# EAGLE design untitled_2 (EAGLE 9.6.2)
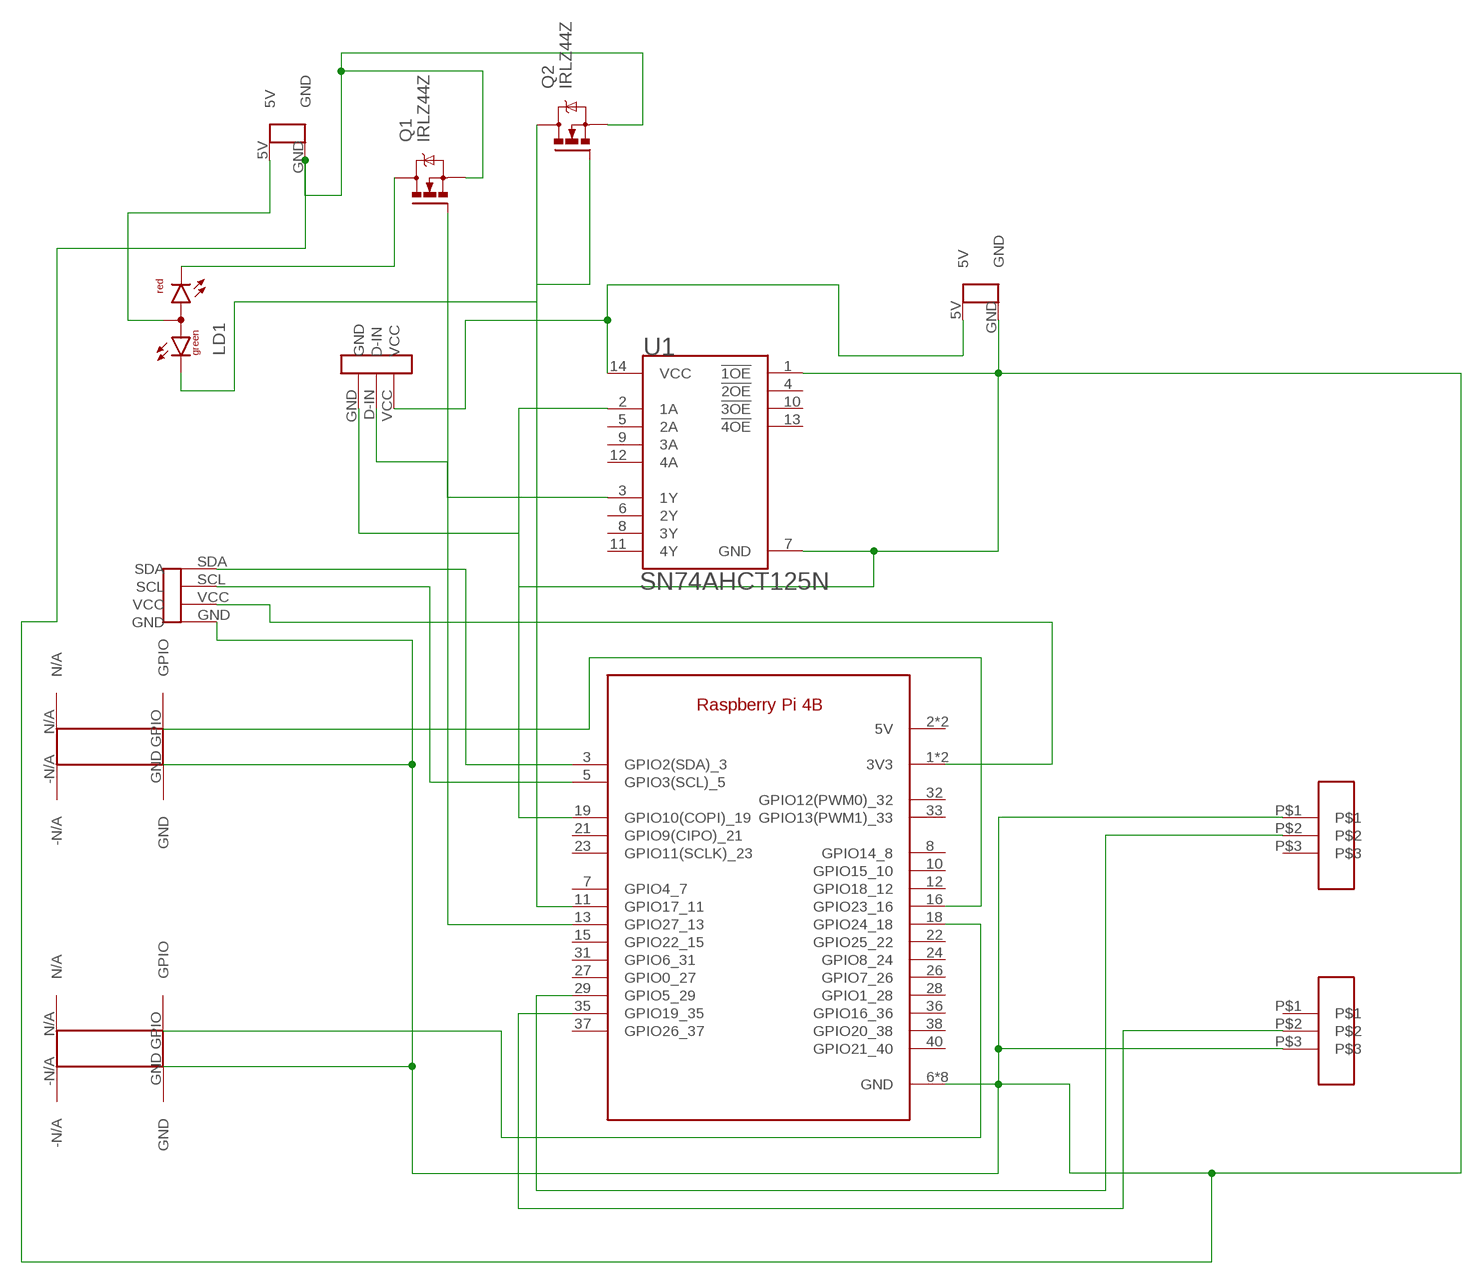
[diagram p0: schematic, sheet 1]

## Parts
LD1  DUOLED-RG-A  [DUOLED-A-5MM]
Q1  IRLZ44Z  [TO220BH]
Q2  IRLZ44Z  [TO220BH]
U1  TEXAS_INSTRUMENTS_SN74AHCT125NTEXAS_INSTRUMENTS_SN74AHCT125N_0_0  [TEXAS_INSTRUMENTS_SN74AHCT125N_0]
U$1  RASPBERRY_PI_4  [RASPI_4B]
U$2  G13-SW  [G13-SW]
U$3  G13-SW  [G13-SW]
U$4  LIGHTSENSOR-PO  [LIGHTSENSOR-IO]
U$5  LED-STRIP-PO  [LED-STRIP-PO]
U$6  G13-BUTTON  [G13-BUTTON]
U$7  G13-BUTTON  [G13-BUTTON]
U$8  G13-BATTERY  [G13-BATTERY]
U$10  G13-BATTERY  [G13-BATTERY]

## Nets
GND: Q1.S Q2.S U1.1(!1OE!) U1.7(GND) U$1.6(GND) U$1.9(GND) U$1.14(GND) U$1.20(GND) U$1.25(GND) U$1.30(GND) U$1.34(GND) U$1.39(GND) U$2.P$1 U$3.P$3 U$4.GND U$5.GND U$6.GND U$7.GND U$8.GND U$10.GND
N$1: U$1.3(GPIO2(SDA)_3) U$4.SDA
N$2: U$1.5(GPIO3(SCL)_5) U$4.SCL
N$3: U$1.1(3V3) U$1.17(3V3) U$4.VCC
N$4: LD1.CR Q1.D
N$5: U$1.16(GPIO23_16) U$6.GPIO
N$6: U$1.18(GPIO24_18) U$7.GPIO
N$7: U$1.29(GPIO5_29) U$2.P$2
N$8: U$1.35(GPIO19_35) U$3.P$2
N$9: U1.2(1A) U$1.19(GPIO10(COPI)_19)
N$10: U1.3(1Y) U$5.D-IN
N$11: U1.14(VCC) U$5.VCC U$8.5V
N$12: LD1.CX(CG) Q2.D
N$13: LD1.A U$10.5V
N$14: Q2.G U$1.11(GPIO17_11)
N$15: Q1.G U$1.13(GPIO27_13)
Unconnected: U1.4(!2OE!) U1.5(2A) U1.6(2Y) U1.8(3Y) U1.9(3A) U1.10(!3OE!) U1.11(4Y) U1.12(4A) U1.13(!4OE!) U$1.2(5V) U$1.4(5V) U$1.7(GPIO4_7) U$1.8(GPIO14_8) U$1.10(GPIO15_10) U$1.12(GPIO18_12) U$1.15(GPIO22_15) U$1.21(GPIO9(CIPO)_21) U$1.22(GPIO25_22) U$1.23(GPIO11(SCLK)_23) U$1.24(GPIO8_24) U$1.26(GPIO7_26) U$1.27(GPIO0_27) U$1.28(GPIO1_28) U$1.31(GPIO6_31) U$1.32(GPIO12(PWM0)_32) U$1.33(GPIO13(PWM1)_33) U$1.36(GPIO16_36) U$1.37(GPIO26_37) U$1.38(GPIO20_38) U$1.40(GPIO21_40) U$2.P$3 U$3.P$1 U$6.-N/A U$6.N/A U$7.-N/A U$7.N/A

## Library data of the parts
LD1 = led:DUOLED-RG-A: DUO LED 2 colors (red/green), 5 mm, round, common Anode www.ligitek.com or other producers.
Q1 Q2 = transistor-power:IRLZ44Z: N-Channel HEXFET® Power MOSFET Logic Level AUTOMOTIVE MOSFET Source: http://www.irf.com/product-info/datasheets/data/irlz44zpbf.pdf
U1 = Texas Instruments - SN74AHCT125N:TEXAS_INSTRUMENTS_SN74AHCT125N: QUADRUPLE BUS BUFFER GATES WITH 3-STATE OUTPUTS; CENTROID_NOT_SPECIFIED: No; DATASHEET: http://www.ti.com/lit/ds/symlink/sn74ahct125.pdf; DIGIKEY_DESCRIPTION: IC BUS BUFFER TRI-ST QD 14DIP; DIGIKEY_PART_NUMBER: 296-4655-5-ND; IPC_LAND_PATTERN_NAME: DIP794W46P254L1930H508Q14; LEAD_FREE: yes; MF: Texas Instruments; MOUSER_PART_NUMBER: 595-SN74AHCT125N; MPN: SN74AHCT125N; PACKAGE: PDIP-14; PREFIX: U; ROHS: yes; TEMPERATURE_RANGE_HIGH: +125°C; TEMPERATURE_RANGE_LOW: -40°C
U$1 = raspberryPi4:RASPBERRY_PI_4
U$2 U$3 = raspberryPi4:G13-SW
U$4 = raspberryPi4:LIGHTSENSOR-PO
U$5 = raspberryPi4:LED-STRIP-PO
U$6 U$7 = raspberryPi4:G13-BUTTON
U$8 U$10 = raspberryPi4:G13-BATTERY

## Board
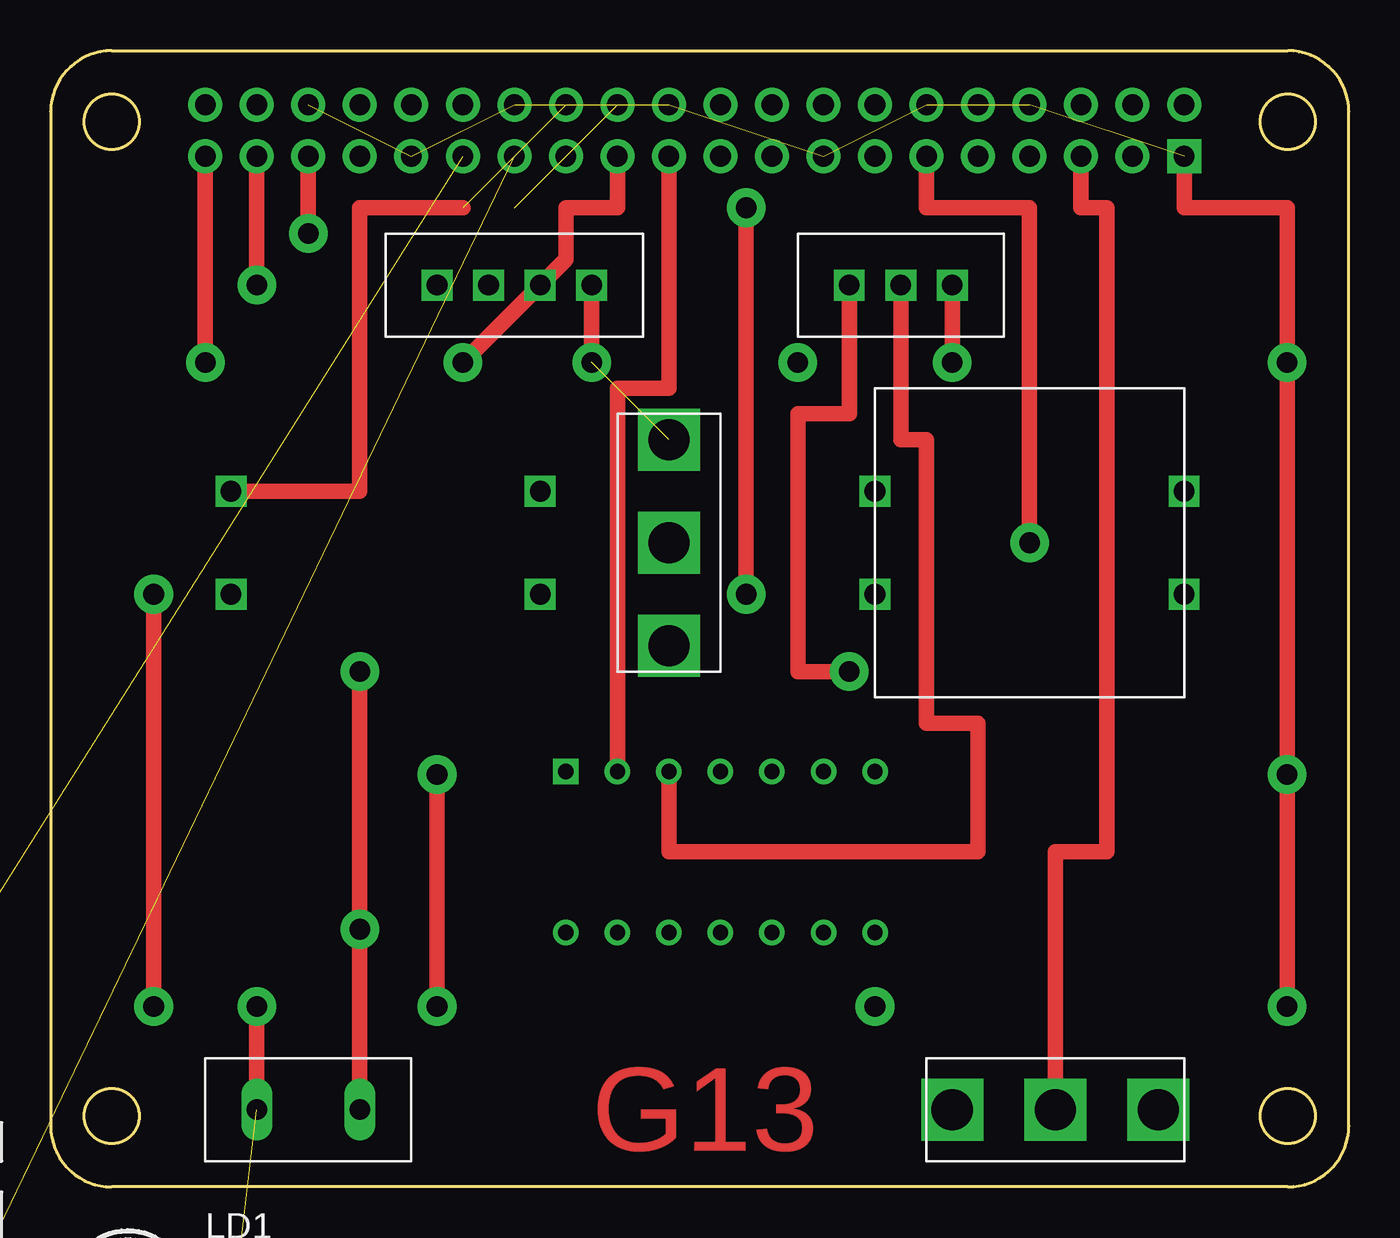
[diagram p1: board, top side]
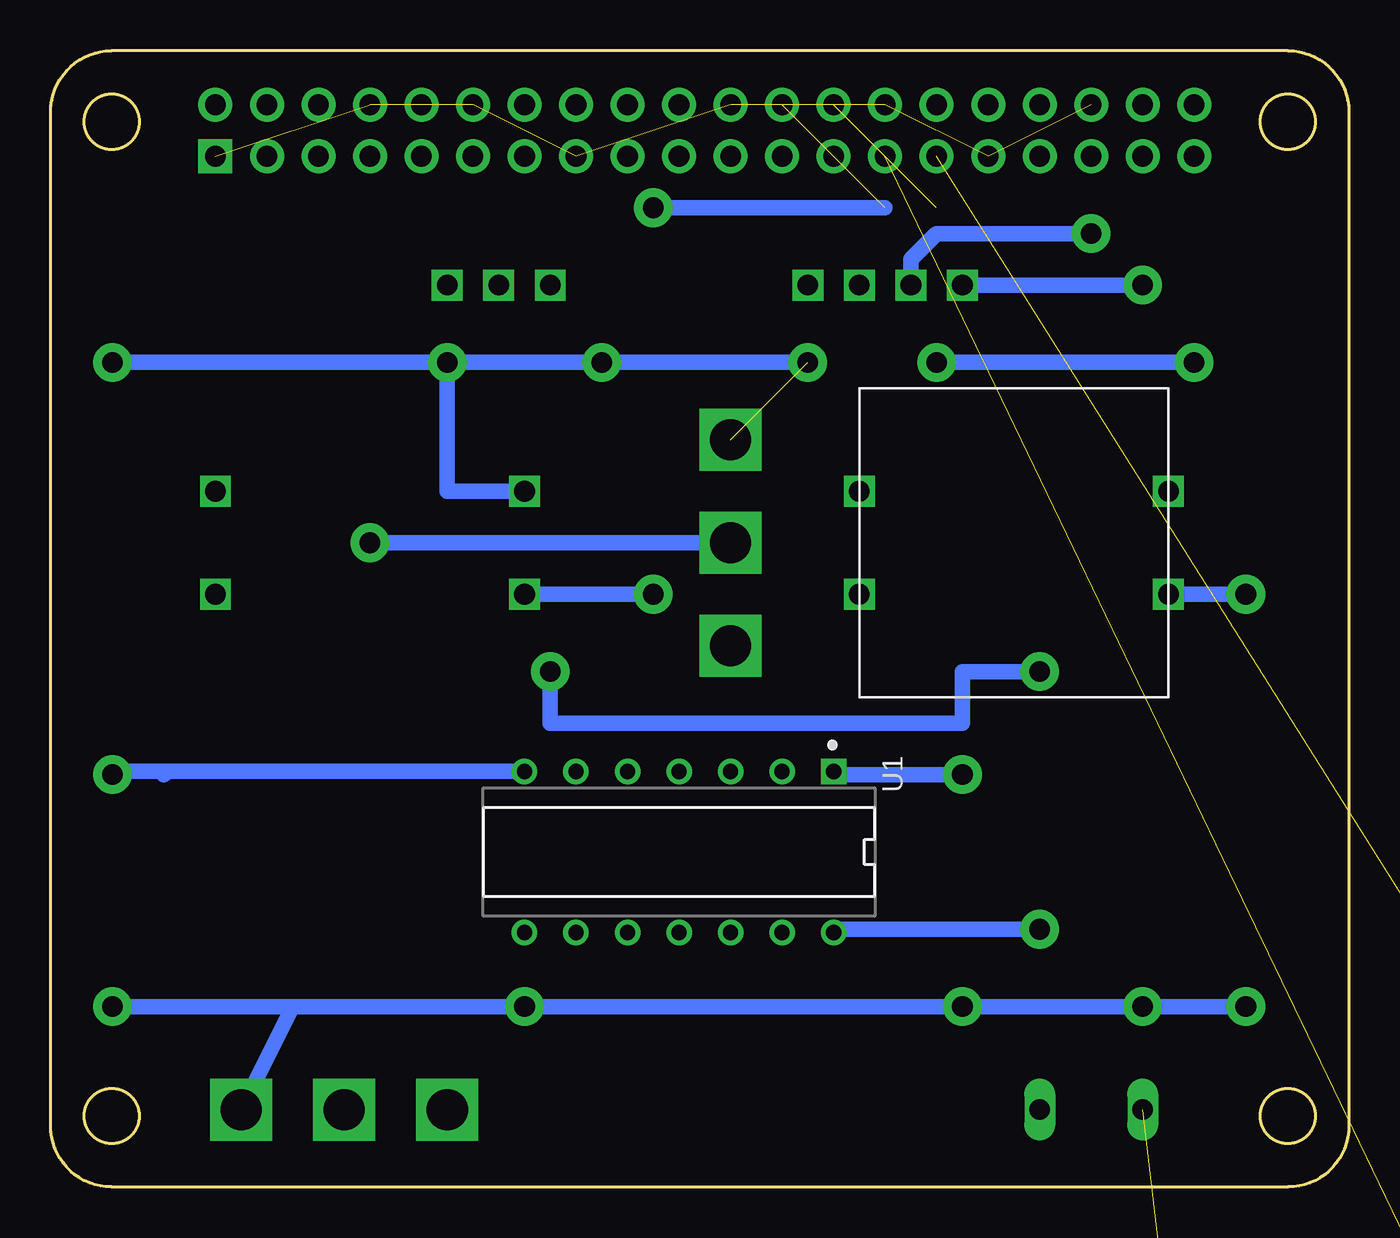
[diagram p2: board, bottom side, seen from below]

Size 64 x 56 mm. Coordinates in mm from the lower left corner, seen from the top.
Outline: 64,3 64,53 arc90 61,56 3,56 arc90 0,53 0,3 arc90 3,0 61,0 arc90 64,3
Outline: circle at 61,52.5 radius 1.35
Outline: circle at 61,3.5 radius 1.35
Outline: circle at 3,52.5 radius 1.35
Outline: circle at 3,3.5 radius 1.35
Copper layers (1*16): Top 0.035mm / dielectric 1.5mm / Bottom 0.035mm
Design rules "default": minimum track width 6mil, minimum drill 0.35mm, track to track 6mil, track to pad 6mil, pad to pad 6mil, via to via 6mil, smd to smd 6mil, copper to edge 40mil, drill to drill 6mil, minimum pad ring 10mil, minimum via ring 8mil, stop-mask expansion 4mil, vias tented up to drill 0mil, thermal gap 10mil

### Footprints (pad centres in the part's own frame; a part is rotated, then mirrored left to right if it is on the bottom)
DUOLED-A-5MM = drill 0.813 long: A 0,0; CR 2.54,0; CX -2.54,0
TO220BH = drill 1.118 long: D 0,-6.35; G -2.54,-6.35; S 2.54,-6.35 | hole 3.302: 0,11.176
TEXAS_INSTRUMENTS_SN74AHCT125N_0 = drill 0.75 pad 1.25 square: 1 -3.97,7.62 | drill 0.75 pad 1.25: 2 -3.97,5.08; 3 -3.97,2.54; 4 -3.97,0; 5 -3.97,-2.54; 6 -3.97,-5.08; 7 -3.97,-7.62; 8 3.97,-7.62; 9 3.97,-5.08; 10 3.97,-2.54; 11 3.97,0; 12 3.97,2.54; 13 3.97,5.08; 14 3.97,7.62
RASPI_4B = drill 1.016 pad 1.676: 1 -24.13,-1.27; 2 -24.13,1.27; 3 -21.59,-1.27; 4 -21.59,1.27; 5 -19.05,-1.27; 6 -19.05,1.27; 7 -16.51,-1.27; 8 -16.51,1.27; 9 -13.97,-1.27; 10 -13.97,1.27; 11 -11.43,-1.27; 12 -11.43,1.27; 13 -8.89,-1.27; 14 -8.89,1.27; 15 -6.35,-1.27; 16 -6.35,1.27; 17 -3.81,-1.27; 18 -3.81,1.27; 19 -1.27,-1.27; 20 -1.27,1.27; 21 1.27,-1.27; 22 1.27,1.27; 23 3.81,-1.27; 24 3.81,1.27; 25 6.35,-1.27; 26 6.35,1.27; 27 8.89,-1.27; 28 8.89,1.27; 29 11.43,-1.27; 30 11.43,1.27; 31 13.97,-1.27; 32 13.97,1.27; 33 16.51,-1.27; 34 16.51,1.27; 35 19.05,-1.27; 36 19.05,1.27; 37 21.59,-1.27; 38 21.59,1.27; 40 24.13,1.27 | drill 1.016 pad 1.676 square: 39 24.13,-1.27
G13-SW = drill 2.032 square: P$1 -5.08,0; P$2 0,0; P$3 5.08,0
LIGHTSENSOR-IO = drill 1.016 square: GND -5.08,0; SCL 0,0; SDA 2.54,0; VCC -2.54,0
LED-STRIP-PO = drill 1.016 square: D-IN 0,0; GND -2.54,0; VCC 2.54,0
G13-BUTTON = drill 1.016 square: -N/A -7.62,-2.54; GND 7.62,-2.54; GPIO 7.62,2.54; N/A -7.62,2.54
G13-BATTERY = drill 1.016 long: 5V -2.54,0; GND 2.54,0

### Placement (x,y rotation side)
LD1  not placed on the board
Q1  not placed on the board
Q2  not placed on the board
U1  33.02,16.51 270 bottom
U$1  31.75,52.07 0 top
U$2  30.48,31.75 270 top
U$3  49.53,3.81 0 top
U$4  21.59,44.45 180 top
U$5  41.91,44.45 180 top
U$6  16.51,31.75 0 bottom
U$7  48.26,31.75 180 top
U$8  12.7,3.81 180 top
U$10  not placed on the board

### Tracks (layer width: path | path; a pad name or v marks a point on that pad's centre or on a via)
GND  (via drill 1.02 pad 1.91)  (11 unrouted)
  Top 0.762: U$1.39 55.88,48.26 60.96,48.26 v60.96,40.64 v60.96,20.32 v60.96,8.89 | U$8.GND v10.16,8.89 | U$4.GND v26.67,40.64 | U$5.GND v44.45,40.64 | v5.08,29.21 v5.08,8.89 | v19.05,20.32 v19.05,8.89
  Bottom 0.762: 52.07,8.89 v60.96,8.89 | 52.07,8.89 v40.64,8.89 v19.05,8.89 v10.16,8.89 v5.08,8.89 | v26.67,40.64 v36.83,40.64 v44.45,40.64 | v44.45,40.64 v60.96,40.64 | U$6.GND v5.08,29.21 | U1.7 58.26,20.48 | 58.26,20.48 58.42,20.32 | 58.26,20.48 60.8,20.48 v60.96,20.32 | U1.1 25.24,20.32 v19.05,20.32 | U$3.P$3 52.07,8.89 | U$7.GND 44.45,34.29 v44.45,40.64
N$1  (via drill 1.02 pad 1.91)
  Top 0.762: v10.16,44.45 U$1.3
  Bottom 0.762: U$4.SDA v10.16,44.45
N$2  (via drill 1.02 pad 1.91)
  Top 0.762: v12.7,46.99 U$1.5
  Bottom 0.762: U$4.SCL 21.59,45.72 20.32,46.99 v12.7,46.99
N$3  (via drill 1.02 pad 1.91)
  Top 0.762: U$1.17 27.94,48.26 25.4,48.26 25.4,45.72 U$4.VCC v20.32,40.64 | U$1.1 v7.62,40.64
  Bottom 0.762: v20.32,40.64 v7.62,40.64
N$4  (1 unrouted)
N$5  (1 unrouted)
  Top 0.762: U$6.GPIO 15.24,34.29 15.24,48.26 20.32,48.26
N$6  (via drill 1.02 pad 1.91)  (1 unrouted)
  Top 0.762: v34.29,29.21 v34.29,48.26
  Bottom 0.762: U$7.GPIO v34.29,29.21 | v34.29,48.26 22.86,48.26
N$7  (via drill 1.02 pad 1.91)
  Top 0.762: v48.26,31.75 48.26,48.26 43.18,48.26 U$1.29
  Bottom 0.762: U$2.P$2 v48.26,31.75
N$8
  Top 0.762: U$3.P$2 49.53,16.51 52.07,16.51 52.07,48.26 50.8,48.26 U$1.35
N$9
  Top 0.762: U1.2 27.94,39.37 30.48,39.37 U$1.19
N$10
  Top 0.762: U1.3 30.48,16.51 45.72,16.51 45.72,22.86 43.18,22.86 43.18,36.83 41.91,36.83 U$5.D-IN
N$11  (via drill 1.02 pad 1.91)
  Top 0.762: U$8.5V v15.24,12.7 v15.24,25.4 | U$5.VCC 39.37,38.1 36.83,38.1 36.83,25.4 v39.37,25.4
  Bottom 0.762: v15.24,12.7 25.24,12.7 U1.14 | v39.37,25.4 39.37,22.86 19.05,22.86 19.05,25.4 v15.24,25.4
N$12  (1 unrouted)
N$13  (1 unrouted)
N$14  (1 unrouted)
N$15  (1 unrouted)

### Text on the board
Top: G13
